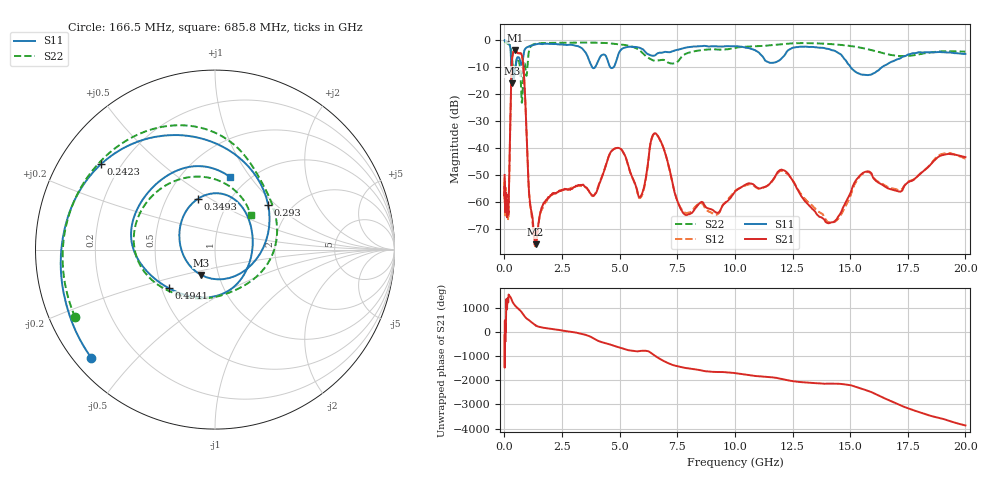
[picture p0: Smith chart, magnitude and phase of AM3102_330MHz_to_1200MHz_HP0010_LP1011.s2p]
! Date/Time: Tue, Sep 11, 2018 5:11 PM
! Network Analyzer: Agilent Technologies E8362B Rev: A.07.50.63
! Sweep from 0.010 to 20.000 GHz, 1601 Points, Sweep Type: LOG
! Power Supply: 4.950 V, 0.001 A
# Hz S DB R 50
!freq MagS11 AngS11 MagS21 AngS21 MagS12 AngS12 MagS22 AngS22
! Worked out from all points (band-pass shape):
!   1601 points, 10 MHz to 20 GHz, reference 50 ohm
!   highest |S21| = -3.57 dB at 449.3 MHz (marker M1); lowest = -75.6 dB at 1.353 GHz (marker M2)
!   |S21| within 3 dB of the highest: 336.2 MHz to 784.3 MHz (448.1 MHz wide, 80 % of centre)
!   lowest |S11| = -15.9 dB at 319.2 MHz (marker M3), VSWR 1.38, Z = 41.3 - j12 ohm
!   |S11| at or under -10 dB: 298.1 MHz to 487.4 MHz (189.3 MHz wide, 48.2 % of centre); 4.599 GHz to 4.725 GHz (125.9 MHz wide, 2.7 % of centre); 15.03 GHz to 16.37 GHz (1.346 GHz wide, 8.57 % of centre)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
!   |S22| runs from -23.1 to -0.3 dB; largest |S21 - S12| = 0.012
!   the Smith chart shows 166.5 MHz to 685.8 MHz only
!   S11 on the Smith chart (normalised r, x): 166.5 MHz: 0.05, -0.38; 242.3 MHz: 0.13, +0.33; 293 MHz: 1.52, +0.90; 349.3 MHz: 0.71, +0.44; 494.1 MHz: 0.54, -0.26; 685.8 MHz: 0.83, +0.81
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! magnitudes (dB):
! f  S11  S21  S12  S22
! 10 MHz  0.0  -49.9  -58.8  -0.3
! 35.55 MHz  0.0  -62.0  -59.8  -0.5
! 126.4 MHz  -0.4  -62.2  -64.6  -1.1
! 166.5 MHz  -0.8  -64.4  -64.8  -1.3
! 242.3 MHz  -2.0  -36.5  -36.6  -1.8
! 293 MHz  -8.2  -15.0  -15.1  -3.5
! 319.2 MHz  -15.9  -8.4  -8.4  -6.0
! 349.3 MHz  -10.5  -5.8  -5.9  -8.1
! 447.2 MHz  -12.3  -3.6  -3.6  -11.0
! 449.3 MHz  -12.2  -3.6  -3.6  -10.9
! 494.1 MHz  -9.5  -3.7  -3.8  -8.8
! 685.8 MHz  -7.7  -4.7  -4.7  -11.2
! 837.2 MHz  -5.0  -11.3  -11.3  -10.8
! 1.353 GHz  -1.5  -75.6  -74.8  -1.2
! 1.59 GHz  -1.3  -62.9  -63.3  -1.0
! 4.855 GHz  -7.6  -39.9  -40.0  -1.3
! 5.652 GHz  -2.4  -52.8  -53.0  -2.6
! 6.612 GHz  -5.0  -34.9  -34.9  -7.5
! 7.845 GHz  -2.7  -64.7  -63.9  -5.0
! 12.09 GHz  -6.1  -48.1  -48.4  -1.3
! 14.07 GHz  -3.2  -67.9  -67.4  -1.3
! 20 GHz  -5.0  -43.3  -43.9  -4.1
